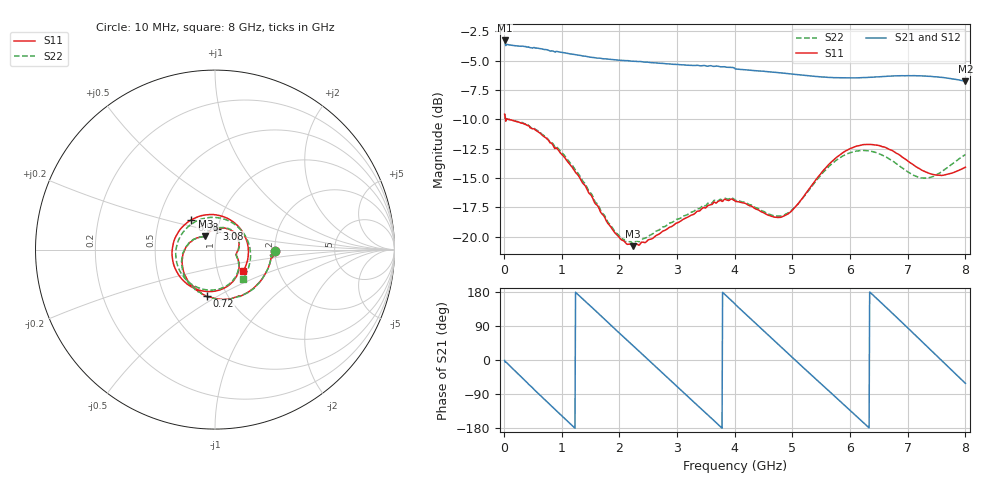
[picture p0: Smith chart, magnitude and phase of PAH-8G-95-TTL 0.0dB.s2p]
! MTS Systemtechnik GmbH
! S-Parameters
! Model: PAH-8G/95-TTL
! Attenuation Step: 0.0dB
! Rohde & Schwarz ZVB8 2Ports - Version 4.11 - 1145.1010k08 SN: 100119
! S2P File Measurements:
! S11 S21 S12 S22
# HZ  S  DB  R  50.00
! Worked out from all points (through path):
!   800 points, 10 MHz to 8 GHz, reference 50 ohm
!   highest |S21| = -3.29 dB at 10 MHz (marker M1); lowest = -6.8 dB at 8 GHz (marker M2)
!   group delay of S21, straight-line fit = 394 ps
!   lowest |S11| = -20.8 dB at 2.24 GHz (marker M3), VSWR 1.20, Z = 44.5 + j6.62 ohm
!   |S11| at or under -10 dB: 25.35 MHz to 38.86 MHz (13.51 MHz wide, 42.1 % of centre); 59.31 MHz to end of sweep
!   |S22| runs from -20.6 to -9.6 dB; largest |S21 - S12| = 0.0066
!   S11 on the Smith chart (normalised r, x): 10 MHz: 1.99, -0.04; 720 MHz: 0.80, -0.45; 3.08 GHz: 0.99, +0.23; 6.98 GHz: 0.73, +0.25; 8 GHz: 1.33, -0.33
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1e7  -9.57 -1.6  -3.29 -1.2  -3.22 -1.1  -9.56 -1.3
4e8  -10.51 -56.0  -3.85 -59.7  -3.83 -59.7  -10.51 -55.9
7.2e8  -11.56 -99.6  -4.06 -106.4  -4.05 -106.5  -11.48 -99.4
1.05e9  -13.26 -142.2  -4.34 -154.1  -4.34 -154.1  -13.10 -142.0
1.35e9  -15.34 -177.2  -4.59 163.1  -4.59 163.1  -15.16 -176.6
1.8e9  -18.87 144.2  -4.87 99.4  -4.87 99.6  -18.75 145.1
2.24e9  -20.82 125.8  -5.05 37.8  -5.04 37.7  -20.62 128.2
2.68e9  -19.80 108.2  -5.22 -24.9  -5.21 -24.8  -19.46 109.7
3.08e9  -18.61 85.6  -5.36 -81.6  -5.36 -81.9  -18.36 86.0
3.6e9  -17.27 55.1  -5.45 -154.3  -5.46 -154.2  -17.15 54.0
4.01e9  -17.01 25.4  -5.72 146.5  -5.72 146.4  -16.93 24.3
4.28e9  -17.39 8.1  -5.83 108.4  -5.83 108.4  -17.30 7.3
4.55e9  -18.10 -5.6  -5.94 70.1  -5.96 70.1  -18.00 -6.4
4.95e9  -17.98 -17.1  -6.12 13.5  -6.14 13.5  -17.91 -18.2
5.34e9  -15.61 -35.8  -6.32 -41.0  -6.34 -41.0  -15.71 -36.3
5.62e9  -13.91 -58.8  -6.43 -79.9  -6.46 -79.9  -14.09 -58.5
5.88e9  -12.83 -85.6  -6.47 -116.1  -6.49 -116.1  -13.12 -84.4
6.29e9  -12.15 -134.1  -6.44 -173.4  -6.46 -173.4  -12.68 -132.1
6.67e9  -12.55 174.8  -6.33 132.5  -6.33 132.7  -13.35 175.7
6.98e9  -13.47 128.2  -6.29 87.7  -6.28 87.7  -14.42 125.5
7.5e9  -14.76 40.4  -6.38 11.6  -6.38 11.5  -14.72 29.8
8e9  -14.09 -37.1  -6.75 -61.7  -6.75 -61.7  -13.01 -46.2
